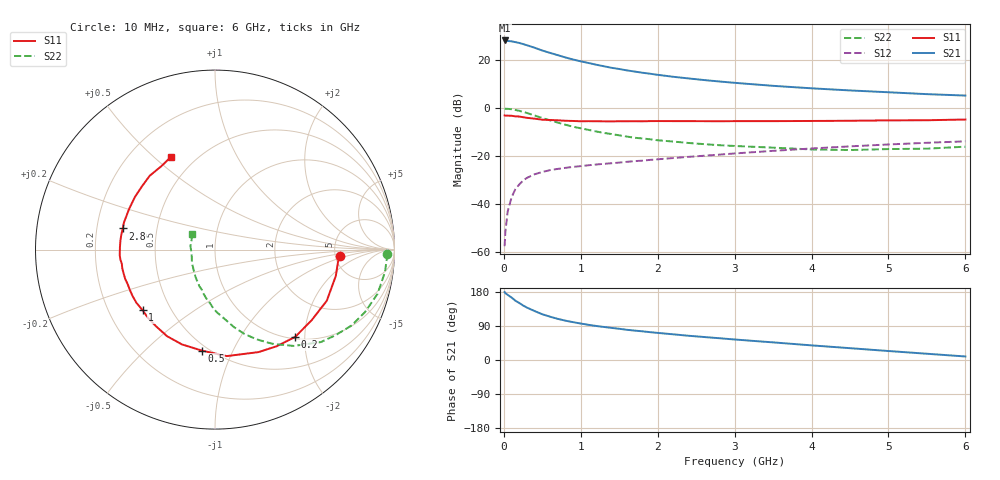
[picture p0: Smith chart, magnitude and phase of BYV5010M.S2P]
! SIEMENS Small Signal Semiconductors
! BFY420
! Si NPN RF SIEGET Grounded Emitter Transistor in MICRO-X
! VCE = 0.5 V  IC = 10 mA
! Common Emitter S-Parameters:  October  1996
# GHz  S  MA  R  50
!  f  S11  S21  S12  S22
! GHz  MAG  ANG  MAG  ANG  MAG  ANG  MAG  ANG
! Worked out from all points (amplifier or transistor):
!   36 points, 10 MHz to 6 GHz, reference 50 ohm
!   highest |S21| = 28.2 dB at 10 MHz (marker M1)
!   |S21| within 3 dB of that: start of sweep to 396.1 MHz
!   unconditionally stable (mu >= 1): 2.238 GHz to end of sweep
!   at 250 MHz: K = 0.21, MSG = 28.5 dB, |S12| = -30.3 dB
!   at 1.4 GHz: K = 0.80, MSG = 19.9 dB, |S12| = -23.1 dB
!   at 6 GHz: K = 1.13, MAG = 7.3 dB, |S12| = -14.0 dB
!   S11 on the Smith chart (normalised r, x): 10 MHz: 5.48, -0.75; 200 MHz: 1.04, -1.79; 500 MHz: 0.46, -0.76; 1 GHz: 0.35, -0.32; 2.8 GHz: 0.31, +0.10; 6 GHz: 0.37, +0.57
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0.01  0.6962 -2.9  25.57 179.3  0.0013 93.6  0.9582 -1.4
0.02  0.6893 -5.2  25.41 176.4  0.0026 87.6  0.9587 -2.9
0.05  0.6888 -12.4  24.96 171.8  0.0069 82.1  0.9552 -7.5
0.1  0.6849 -24.6  24.52 164.9  0.0135 78.8  0.9385 -15.2
0.15  0.667 -36.1  23.61 156.5  0.0202 73.1  0.9054 -22.6
0.2  0.6604 -47.4  22.69 150.6  0.0252 68.9  0.871 -29.0
0.25  0.6389 -57.4  21.54 143.9  0.0305 62.9  0.8235 -35.4
0.3  0.6204 -67.0  20.33 138.3  0.0346 61.0  0.7835 -41.1
0.4  0.5969 -83.7  18.02 129.2  0.0412 53.9  0.6937 -50.7
0.5  0.5672 -97.6  15.76 120.7  0.046 49.6  0.6149 -58.6
0.6  0.5594 -109.3  14.08 114.3  0.0502 46.9  0.5496 -65.3
0.7  0.5515 -119.0  12.63 108.6  0.0533 45.3  0.4944 -71.1
0.8  0.539 -127.4  11.31 103.8  0.0561 42.9  0.4453 -76.2
1  0.5261 -140.1  9.368 96.2  0.0609 41.7  0.3746 -84.2
1.1  0.5288 -146.0  8.661 92.8  0.0635 40.9  0.3478 -88.6
1.6  0.5261 -165.6  6.064 79.7  0.0749 40.2  0.2522 -104.9
2.2  0.5299 178.7  4.467 67.8  0.0897 39.6  0.1985 -120.6
2.8  0.5268 167.1  3.564 57.5  0.1058 37.9  0.1665 -135.2
3.5  0.5294 154.8  2.888 46.5  0.1269 34.8  0.148 -150.3
4.5  0.5386 139.0  2.316 31.2  0.1575 27.4  0.132 -172.9
5.5  0.5528 122.6  1.937 16.5  0.187 18.5  0.1409 157.8
6  0.5721 115.4  1.809 9.3  0.2005 13.8  0.1553 145.9
